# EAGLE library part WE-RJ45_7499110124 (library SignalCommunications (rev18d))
Order Code 7499110124 Design THT xBase-T 10/100/1000 Base-T Ports 1x1 Application Standard Tab Position UP LED (Left-Right) GREEN/YELLOW-GREEN EMI Fingers No Details see: http://katalog.we-online.de/en/pbs/WE-LAN_RJ45/7499110124? Updated by Yingchun Shan 2016-08-29 2016(C) Würth Elektronik
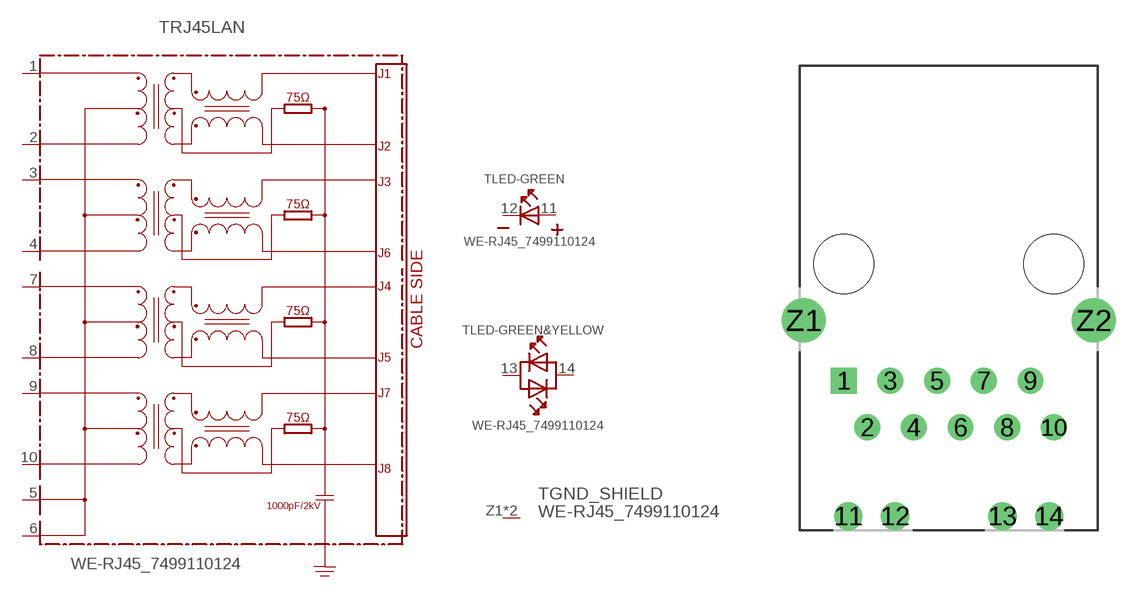
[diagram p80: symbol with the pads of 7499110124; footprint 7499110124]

Designator prefix T; gates RJ45LAN=7499110124 LED-GREEN=LED2PIN LED-GREEN&YELLOW=LED-DUAL-1 GND_SHIELD=GNDPIN

## WE-RJ45_7499110124 (COMPANY-URL: http://www.we-online.de; CREATED-BY: Christin Zierenner; CREATED-DATE: AUG 2012; DATASHEET-URL: http://katalog.we-online.de/kataloge/eisos/media/pdf/7499110124.pdf; MANUFACTURER: Würth Elektronik eiSos GmbH)  [7499110124]
1  RJ45LAN:1
2  RJ45LAN:2
3  RJ45LAN:3
4  RJ45LAN:4
5  RJ45LAN:5
6  RJ45LAN:6
7  RJ45LAN:7
8  RJ45LAN:8
9  RJ45LAN:9
10  RJ45LAN:10
11  LED-GREEN:A  pas
12  LED-GREEN:K  pas
13  LED-GREEN&YELLOW:AK1  pas
14  LED-GREEN&YELLOW:AK2  pas
Z1  GND_SHIELD:GND  pwr
Z2  GND_SHIELD:GND  pwr

## Footprint 7499110124 (pad centres in mm)
MAX HEIGHT=13.50mm PORTS----1X1 LED --YES
drill 0.9 square: 1 -5.715,-6.35
drill 0.9: 2 -4.445,-8.89; 3 -3.175,-6.35; 4 -1.905,-8.89; 5 -0.635,-6.35; 6 0.635,-8.89; 7 1.905,-6.35; 8 3.175,-8.89; 9 4.445,-6.35; 10 5.715,-8.89
drill 1.02: 11 -5.465,-13.72; 12 -2.925,-13.72; 13 2.925,-13.72; 14 5.465,-13.72
drill 1.6: Z1 -7.9,-3.05; Z2 7.9,-3.05
hole 3.25 at 5.715,0
hole 3.25 at -5.715,0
